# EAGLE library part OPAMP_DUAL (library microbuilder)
Dual Op-Amp MSOP8 - 0.65mm Pitch Manuf. ID Slew Rate Gain Bandwidth Prod. -3dB Bandwidth Current Input Bias Voltage Input Offset Supply - Single Supply - Dual Digikey Mouser EL5236IYZ-T7 128V/µs 300MHz 250MHz 6.5µA 100µV 5-12V +/-2.5-6V EL5236IYZ-T7TR-ND --
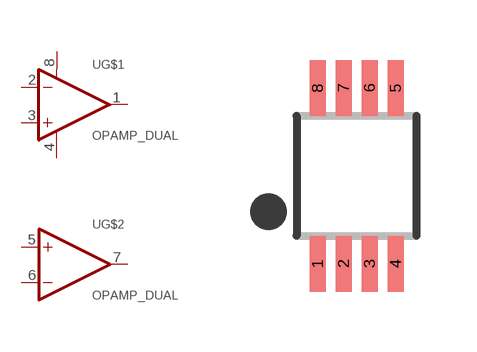
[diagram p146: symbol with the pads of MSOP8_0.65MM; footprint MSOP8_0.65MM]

Designator prefix U; gates G$1=OPAMP+- G$2=OPAMP

## OPAMP_DUALMSOP8_65  [MSOP8_0.65MM]
1  G$1:OUT  out
2  G$1:-IN  in
3  G$1:+IN  in
4  G$1:V-  pwr
5  G$2:+IN  in
6  G$2:-IN  in
7  G$2:OUT  out
8  G$1:V+  pwr

## Footprint MSOP8_0.65MM (pad centres in mm)
Source: http://www.intersil.com/data/fn/fn7833.pdf
smd 0.4 x 1.4: 1 -0.975,-2.2; 2 -0.325,-2.2; 3 0.325,-2.2; 4 0.975,-2.2; 5 0.975,2.2; 6 0.325,2.2; 7 -0.325,2.2; 8 -0.975,2.2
